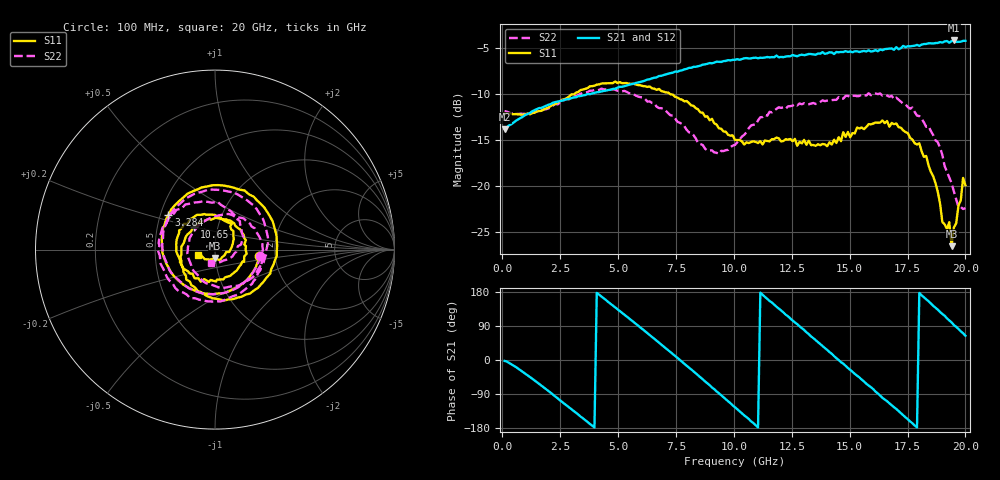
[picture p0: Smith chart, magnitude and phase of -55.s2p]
!Agilent Technologies,N5230C,MY49001569,A.09.33.09
!Agilent N5230C: A.09.33.09
!Date: Tuesday, July 28, 2015 16:38:44
!Correction: S11(Full 2 Port(1,2))
!S21(Full 2 Port(1,2))
!S12(Full 2 Port(1,2))
!S22(Full 2 Port(1,2))
!S2P File: Measurements: S11, S21, S12, S22:
# Hz S  dB  R 50
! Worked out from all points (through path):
!   201 points, 100 MHz to 20 GHz, reference 50 ohm
!   highest |S21| = -4.23 dB at 19.5 GHz (marker M1); lowest = -13.8 dB at 100 MHz (marker M2)
!   group delay of S21, straight-line fit = 143 ps
!   lowest |S11| = -26.5 dB at 19.4 GHz (marker M3), VSWR 1.10, Z = 49.7 - j4.71 ohm
!   |S11| at or under -10 dB: start of sweep to 3.129 GHz; 7.23 GHz to end of sweep
!   |S22| runs from -22.5 to -9.4 dB; largest |S21 - S12| = 0.032
!   S11 on the Smith chart (normalised r, x): 100 MHz: 1.64, -0.13; 3.284 GHz: 0.55, +0.24; 10.65 GHz: 0.77, +0.20; 20 GHz: 0.82, -0.05
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1e8  -12.12 -8.3  -13.84 -2.5  -13.81 -1.3  -11.88 -7.7
1.493e9  -11.92 -106.1  -11.67 -58.3  -11.70 -58.8  -11.91 -104.5
3.284e9  -9.81 143.5  -10.26 -144.0  -10.32 -144.6  -10.14 146.6
3.483e9  -9.55 132.2  -10.18 -153.7  -10.19 -154.0  -9.89 136.0
4.876e9  -8.68 63.4  -9.46 138.9  -9.41 138.7  -9.58 67.3
5.871e9  -9.07 16.9  -8.78 90.5  -8.79 90.1  -10.32 19.8
6.7665e9  -9.48 -23.5  -8.09 46.0  -8.13 45.5  -11.56 -24.9
8.259e9  -11.32 -92.5  -7.09 -30.0  -7.15 -30.5  -14.48 -110.7
9.254e9  -13.33 -144.8  -6.53 -82.9  -6.59 -83.0  -16.40 174.1
1.005e10  -15.00 167.9  -6.32 -124.6  -6.31 -125.0  -15.54 113.3
1.0647e10  -15.34 132.4  -6.19 -155.8  -6.26 -156.4  -13.72 73.9
1.1443e10  -15.12 82.7  -6.03 161.7  -6.10 161.8  -12.38 32.6
1.2239e10  -14.92 39.2  -5.98 119.6  -5.93 120.1  -11.63 -5.0
1.3433e10  -15.56 -30.7  -5.74 57.6  -5.81 57.0  -11.00 -62.7
1.4826e10  -14.67 -119.8  -5.39 -15.5  -5.52 -16.5  -10.24 -131.0
1.5821e10  -13.30 -177.1  -5.30 -67.4  -5.41 -68.8  -9.95 -179.0
1.67165e10  -13.58 136.4  -5.12 -114.2  -5.20 -114.7  -10.33 138.7
1.79105e10  -15.49 70.2  -4.71 -177.8  -4.68 -178.4  -12.38 75.8
1.8607e10  -18.93 25.9  -4.56 143.2  -4.52 142.9  -14.48 38.3
1.9403e10  -26.51 -90.4  -4.31 99.2  -4.42 98.0  -19.68 -22.4
1.95025e10  -24.49 -112.3  -4.23 92.3  -4.40 92.2  -20.57 -31.0
2e10  -19.91 -164.1  -4.27 64.0  -4.46 63.3  -22.38 -105.3
